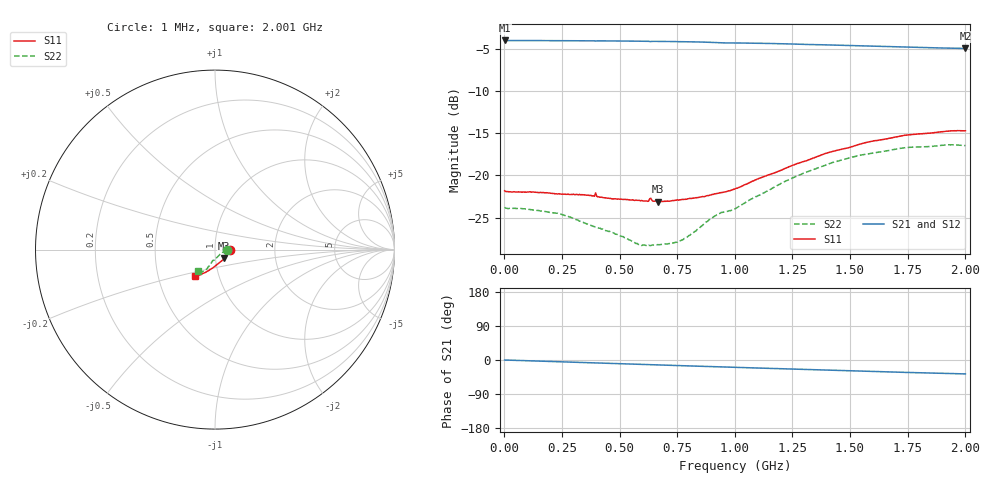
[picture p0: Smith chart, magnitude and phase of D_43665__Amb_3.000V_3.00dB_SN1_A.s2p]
! device id: 43665_
! dir: \\malibu\benchdata\1_engineers\tn_data\43665_75ohm\new\sparar\43665_\amb\3p000v\3p00db
! Serial: 1
! Insertion: A
! Temp: Amb
! VDD: 3.000V
! Attenuation Step: 3.00dB
! IDD: 1.453558e+00mA
! FILE NAME
! DATE 03-27-2009 08:34:06
! CORRECTED  DATA
#  Hz  S  RI  R  75
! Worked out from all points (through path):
!   401 points, 1 MHz to 2.001 GHz, reference 75 ohm
!   highest |S21| = -4.00 dB at 1 MHz (marker M1); lowest = -4.9 dB at 2.001 GHz (marker M2)
!   group delay of S21, straight-line fit = 52 ps
!   lowest |S11| = -23.1 dB at 666 MHz (marker M3), VSWR 1.15, Z = 82.8 - j7.86 ohm
!   |S11| at or under -10 dB: start of sweep to end of sweep
!   |S22| runs from -28.4 to -16.4 dB; largest |S21 - S12| = 0.0031
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1000000  0.0811 -0.00136  0.6312 -0.000953  0.6318 -0.00102  0.0647 -0.00072
9.6e7  0.0794 -0.00491  0.63 -0.0201  0.6302 -0.02  0.0634 -0.00133
2.26e8  0.077 -0.012  0.6278 -0.0471  0.6281 -0.047  0.0595 -0.00456
3.36e8  0.0745 -0.0195  0.6246 -0.0703  0.6249 -0.07  0.0526 -0.00709
5.06e8  0.065 -0.0318  0.6177 -0.1055  0.6177 -0.1056  0.0405 -0.0163
5.86e8  0.0596 -0.039  0.6127 -0.1217  0.6126 -0.1219  0.0323 -0.022
6.41e8  0.0555 -0.0443  0.6089 -0.1329  0.6093 -0.1331  0.0278 -0.0269
6.66e8  0.0516 -0.0473  0.6079 -0.1381  0.6078 -0.1382  0.0261 -0.0289
6.71e8  0.0513 -0.0478  0.6075 -0.1391  0.6074 -0.1393  0.0253 -0.0294
7.61e8  0.0427 -0.0576  0.6006 -0.1579  0.6006 -0.1579  0.0162 -0.0376
7.96e8  0.0388 -0.0615  0.5976 -0.1651  0.5974 -0.1653  0.0124 -0.0416
9.21e8  0.021 -0.0752  0.5828 -0.19  0.583 -0.1897  -0.00269 -0.0582
1.001e9  0.0124 -0.0823  0.5758 -0.2012  0.5761 -0.2012  -0.0137 -0.0619
1.211e9  -0.0205 -0.107  0.5537 -0.2397  0.5543 -0.2401  -0.0291 -0.0866
1.336e9  -0.0403 -0.1194  0.5376 -0.2588  0.5384 -0.2594  -0.0407 -0.0999
1.401e9  -0.0508 -0.1261  0.5293 -0.2694  0.53 -0.2704  -0.0444 -0.1073
1.511e9  -0.0669 -0.1325  0.5146 -0.2835  0.515 -0.2849  -0.0566 -0.1157
1.586e9  -0.0774 -0.1387  0.5051 -0.2935  0.5053 -0.2954  -0.0613 -0.12
1.671e9  -0.0872 -0.1413  0.4942 -0.3036  0.4935 -0.3053  -0.0692 -0.1224
1.741e9  -0.095 -0.1448  0.4852 -0.3116  0.4846 -0.3135  -0.0747 -0.1258
1.911e9  -0.108 -0.1469  0.4642 -0.3294  0.463 -0.3298  -0.0882 -0.1233
2.001e9  -0.1117 -0.1462  0.4538 -0.3383  0.451 -0.3397  -0.092 -0.1188
